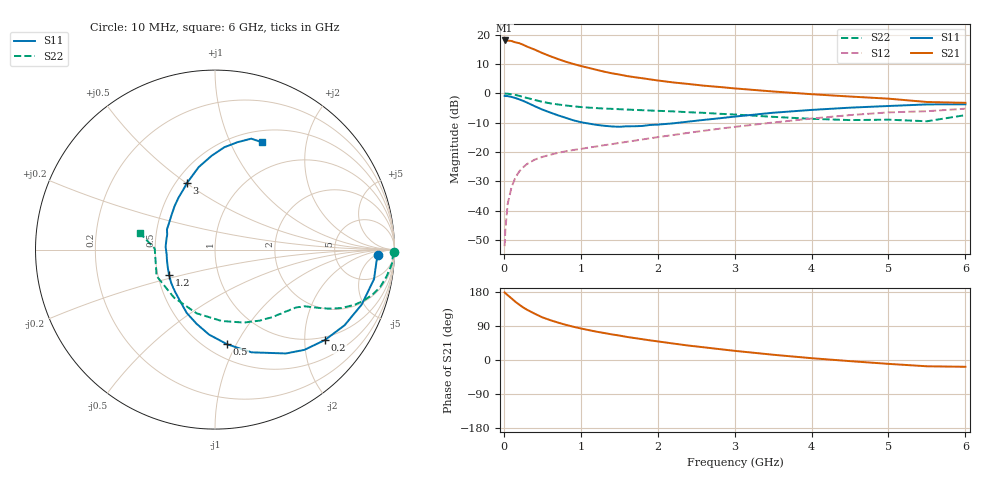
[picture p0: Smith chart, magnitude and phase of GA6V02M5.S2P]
! Infineon Technologies  Discrete & RF Semiconductors
! BF775
! Si NPN RF Bipolar Junction Transistor in SOT23
! VCE = 6 V  IC = 2.5 mA
! Common Emitter S-Parameters:  May  1996
# GHz  S  MA  R  50
!  f  S11  S21  S12  S22
! GHz  MAG  ANG  MAG  ANG  MAG  ANG  MAG  ANG
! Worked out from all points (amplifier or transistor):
!   36 points, 10 MHz to 6 GHz, reference 50 ohm
!   highest |S21| = 18.1 dB at 10 MHz (marker M1)
!   |S21| within 3 dB of that: start of sweep to 389.2 MHz
!   unconditionally stable (mu >= 1): 1.116 GHz to 3.326 GHz
!   at 250 MHz: K = 0.32, MSG = 20.9 dB, |S12| = -25.2 dB
!   at 1.4 GHz: K = 1.10, MAG = 10.1 dB, |S12| = -17.3 dB
!   at 6 GHz: K = 0.94, MSG = 1.0 dB, |S12| = -5.2 dB
!   S11 on the Smith chart (normalised r, x): 10 MHz: 18, -7; 200 MHz: 0.92, -2.50; 500 MHz: 0.63, -0.92; 1.2 GHz: 0.57, -0.17; 3 GHz: 0.57, +0.50; 6 GHz: 0.63, +1.32
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0.01  0.9088 -2.0  7.996 178.4  0.0025 91.8  0.9978 -0.9
0.02  0.9024 -4.1  7.845 176.2  0.0048 85.1  0.9919 -1.8
0.05  0.9012 -10.5  7.955 171.1  0.0131 85.1  0.9895 -4.5
0.1  0.8731 -20.5  7.827 162.6  0.0254 79.2  0.9681 -8.8
0.15  0.8359 -30.3  7.431 153.7  0.0368 72.9  0.9438 -12.8
0.2  0.7933 -39.4  7.181 146.1  0.0468 68.6  0.9101 -16.2
0.25  0.7483 -48.3  6.767 138.9  0.055 64.2  0.8729 -19.1
0.3  0.7005 -55.7  6.297 132.8  0.0626 61.7  0.8394 -21.4
0.4  0.6076 -70.4  5.588 122.3  0.0744 56.2  0.7761 -24.8
0.5  0.5316 -82.7  4.885 112.6  0.0829 53.0  0.7199 -27.2
0.6  0.4747 -94.0  4.327 105.4  0.0901 51.0  0.6797 -28.7
0.8  0.3863 -114.1  3.486 93.1  0.1031 49.2  0.625 -30.8
0.9  0.3496 -123.2  3.188 87.9  0.1086 49.0  0.6042 -31.7
1.1  0.3073 -142.4  2.73 79.0  0.1195 49.7  0.574 -33.8
1.2  0.292 -151.4  2.534 74.9  0.1247 50.1  0.563 -34.7
1.6  0.2756 176.8  1.98 60.9  0.15 51.1  0.5319 -39.7
2.2  0.3095 141.5  1.54 43.5  0.1957 51.9  0.4947 -49.5
3  0.4031 112.7  1.219 24.2  0.2694 48.4  0.4377 -68.3
3.5  0.4691 101.1  1.08 13.9  0.3197 44.0  0.3995 -84.7
4.5  0.5726 84.8  0.886 -3.0  0.4279 32.2  0.3518 -130.4
5.5  0.6503 71.9  0.715 -16.6  0.4982 16.2  0.3359 179.0
6  0.6527 66.6  0.692 -17.9  0.5499 11.8  0.4274 167.7
